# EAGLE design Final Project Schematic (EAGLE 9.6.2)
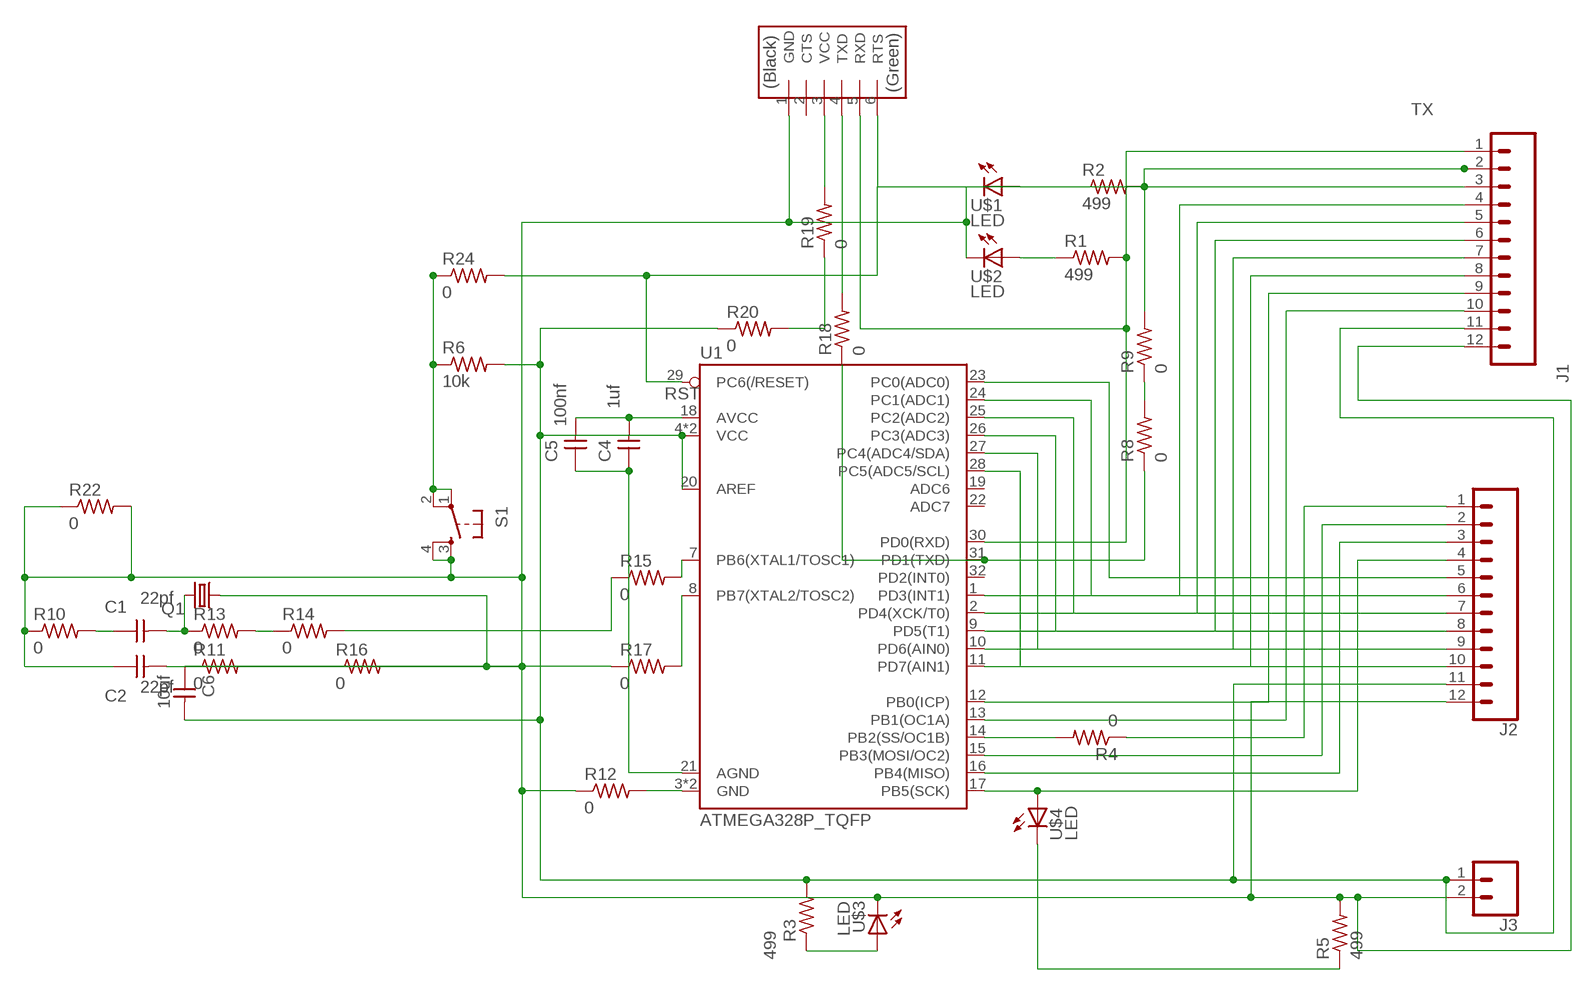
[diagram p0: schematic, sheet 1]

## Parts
C1  22pf  CAP_UNPOLARIZED  [C1206]
C2  22pf  CAP_UNPOLARIZED  [C1206]
C4  1uf  CAP_UNPOLARIZED  [C1206]
C5  100nf  CAP_UNPOLARIZED  [C1206]
C6  10uf  CAP_UNPOLARIZED  [C1206]
J1  CONN_12LONGPADS  [1X12_LONGPADS]
J2  CONN_12LONGPADS  [1X12_LONGPADS]
J3  CONN_02PTH3  [1X02_LONGPADS]
Q1  CRYSTALSM49  [SM49]
R1  499  R1206  [R1206]
R2  499  R1206  [R1206]
R3  499  R1206  [R1206]
R4  0  R1206FAB  [R1206FAB]
R5  499  R1206  [R1206]
R6  10k  R1206  [R1206]
R8  0  R1206FAB  [R1206FAB]
R9  0  R1206FAB  [R1206FAB]
R10  0  R1206FAB  [R1206FAB]
R11  0  R1206FAB  [R1206FAB]
R12  0  R1206FAB  [R1206FAB]
R13  0  R1206FAB  [R1206FAB]
R14  0  R1206FAB  [R1206FAB]
R15  0  R1206FAB  [R1206FAB]
R16  0  R1206FAB  [R1206FAB]
R17  0  R1206FAB  [R1206FAB]
R18  0  R1206FAB  [R1206FAB]
R19  0  R1206FAB  [R1206FAB]
R20  0  R1206FAB  [R1206FAB]
R22  0  R1206FAB  [R1206FAB]
R24  0  R1206FAB  [R1206FAB]
S1  SW_SWITCH_TACTILE_6MM6MM_SWITCH  [6MM_SWITCH]
U1  ATMEGA328P_TQFP  [TQFP32-08]
U$1  LED  [LED1206]
U$2  LED  [LED1206]
U$3  LED  [LED1206]
U$4  LED  [LED1206]
U$5  CONN_06_FTDI-SMD-HEADER  [1X06SMD]

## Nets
3: J1.4 U1.1(PD3(INT1))
4: J1.5 U1.2(PD4(XCK/T0))
5: J1.6 U1.9(PD5(T1))
6: J1.7 U1.10(PD6(AIN0))
7: J1.8 U1.11(PD7(AIN1))
8: J1.9 U1.12(PB0(ICP))
9: J1.10 U1.13(PB1(OC1A))
10: J2.1 R4.1
11: J2.2 U1.15(PB3(MOSI/OC2))
12: J2.3 U1.16(PB4(MISO))
13: J2.4 U1.17(PB5(SCK)) U$4.1(A)
A0: J2.5 U1.23(PC0(ADC0))
A1: J2.6 U1.24(PC1(ADC1))
A2: J2.7 U1.25(PC2(ADC2))
A3: J2.8 U1.26(PC3(ADC3))
A4: J2.9 U1.27(PC4(ADC4/SDA))
A5: J2.10 U1.28(PC5(ADC5/SCL))
GND [through pad 2]: C1.1 C2.1 C2.2 C4.1 C5.1 C6.1 J1.12 J2.12 J3.2 Q1.1 R5.2 R10.1 R10.2 R11.1 R12.1 R12.2 R22.1 R22.2 S1.3(S) S1.4(S1) U1.3(GND) U1.5(GND) U1.21(AGND) U$1.2(C) U$2.2(C) U$3.2(C) U$5.1(GND)
N$1: R4.2 U1.14(PB2(SS/OC1B))
N$2: R2.1 U$1.1(A)
N$18: R6.1 R24.1 S1.1(P) S1.2(P1)
N$25: R18.2 U$5.4(TXD)
N$26: R3.1 U$3.1(A)
N$27: C1.2 Q1.2 R13.1
N$28: R17.2 U1.8(PB7(XTAL2/TOSC2))
N$29: R5.1 U$4.2(C)
N$39: R15.2 U1.7(PB6(XTAL1/TOSC1))
N$40: R13.2 R14.1
N$41: R11.2 R16.1 R16.2 R17.1
N$42: R14.2 R15.1
RST [through pad 2]: J1.3 R24.2 U1.29(PC6(/RESET)) U$5.6(RTS)
RX: J1.1 R1.1 R1.2 U1.30(PD0(RXD)) U$2.1(A) U$5.5(RXD)
TX: J1.2 R2.2 R8.1 R8.2 R9.1 R9.2 R18.1 U1.31(PD1(TXD))
VCC [through pad 2]: C4.2 C5.2 C6.2 J1.11 J2.11 J3.1 R3.2 R6.2 R19.1 R19.2 R20.1 R20.2 U1.4(VCC) U1.6(VCC) U1.18(AVCC) U1.20(AREF) U$5.3(VCC)
Unconnected: U1.19(ADC6) U1.22(ADC7) U1.32(PD2(INT0)) U$5.2(CTS)

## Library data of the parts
C1 C2 C5 C6 = eagle_fab:CAP_UNPOLARIZED
C4 = eagle_fab:CAP_UNPOLARIZED; SPICEPREFIX: C
J1 J2 = SparkFun-Connectors:CONN_12: Multi connection point. Often used as Generic Header-pin footprint for 0.1 inch spaced/style header connections On any of the 0.1 inch spaced packages, you can populate with these: Break Away Headers - Straight (PRT-00116) Break Away Male Headers - Right Angle (PRT-00553) Female Headers (PRT-00115)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
J3 = SparkFun-Connectors:CONN_02: Multi connection point. Often used as Generic Header-pin footprint for 0.1 inch spaced/style header connections
Q1 = crystal:CRYSTAL: CRYSTAL; OC_FARNELL: unknown; OC_NEWARK: unknown
R1-R6 R8-R20 = eagle_fab:R: Resistor (US Symbol)
R22 R24 = fab_new:R: Resistor (US Symbol)
S1 = eagle_fab:SW_SWITCH_TACTILE_6MM: OMRON SWITCH
U1 = SparkFun-IC-Microcontroller:ATMEGA328P_TQFP: Popular 328P in QFP Storefront component: ATmega328 - TQFP (COM-13448) Datasheet SparkFun Products SparkFun RedBoard - Programmed with Arduino (DEV-12757) Arduino Pro Mini 328 - 5V/16MHz (DEV-11113) Arduino Pro Mini 328 - 3.3V/8MHz (DEV-11114) SparkFun OpenLog (DEV-13712) SparkFun MicroView - OLED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; PROD_ID: IC-09069
U$1-U$4 = eagle_fab:LED: LED
U$5 = eagle_fab:CONN_06_FTDI-SMD-HEADER

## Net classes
0 default: width 0.406 mm
1 ground: width 0.559 mm
2 vcc: width 0.559 mm
3 through pad: width 0.33 mm
4 bubble: width 0.229 mm
5 through pad 2: width 0.279 mm

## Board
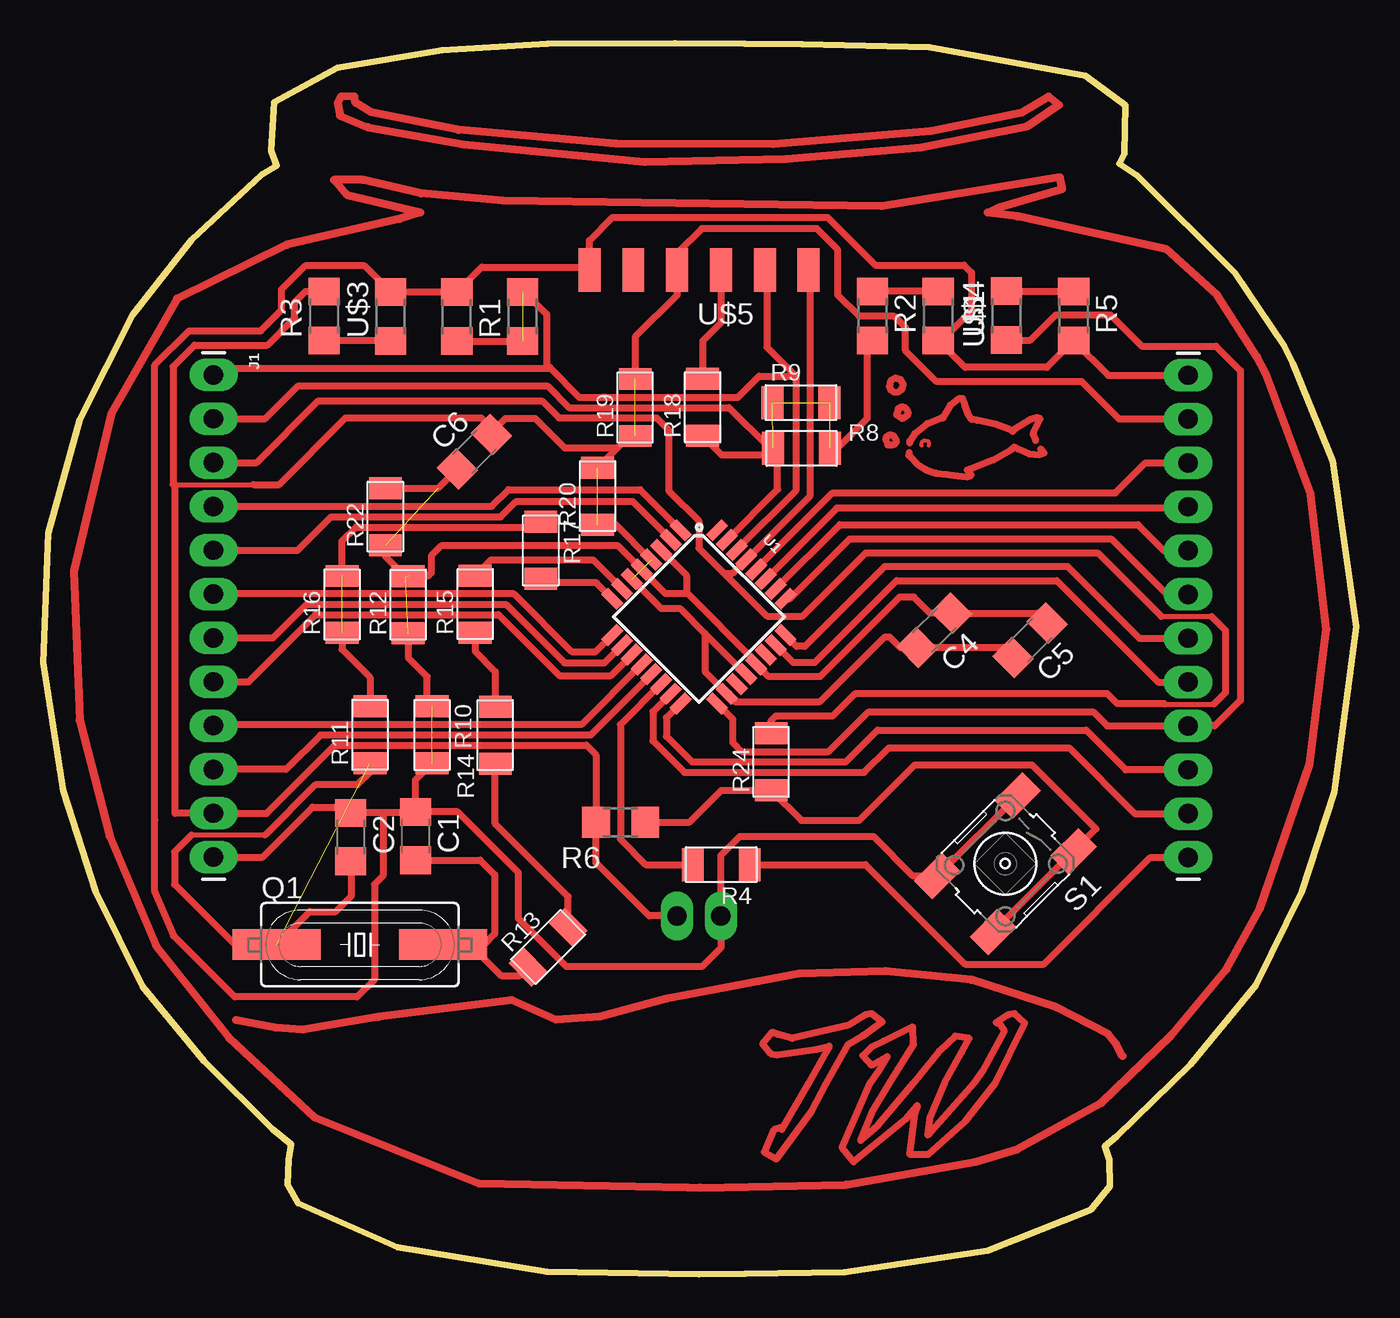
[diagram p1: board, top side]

Size 76.12 x 71.34 mm. Coordinates in mm from the lower left corner, seen from the top.
Outline: 40.67,71.3 36.62,71.34 29.24,71.32 23.12,70.94 17.08,69.91 13.39,67.93 13.22,65.12 13.55,64.24 12.66,63.71 8.62,59.94 5.19,55.61 2.12,49.51 0.29,42.93 0,35.44 1.15,28.03 3.04,22.18 5.77,16.68 9.33,12.35 13.31,8.41 14.38,7.53 14.24,6.64 14.16,5.19 14.77,4.13 20.53,1.58 29.21,0.16 38.03,0 40.67,0.04 46.44,0.14 54.74,1.38 60.74,3.76 61.83,5.1 61.8,6.64 61.55,7.42 62.22,8 66.51,12.14 70.29,16.74 72.96,22.17 74.84,27.93 76.12,37.52 74.75,47.11 72.44,52.79 71.92,53.84 69.07,58.03 63.42,63.66 62.38,64.35 62.68,64.93 62.73,67.74 60.4,69.45 51.37,71.1 43.99,71.27 40.67,71.3
Copper layers (1*16): Top 0.035mm / dielectric 1.5mm / Bottom 0.035mm
Design rules "OthermillDRC_30_deg_v2": minimum track width 6mil, minimum drill 0.8mm, track to track 6mil, track to pad 6mil, pad to pad 6mil, via to via 6mil, smd to smd 0mil, copper to edge 0mil, drill to drill 6mil, minimum pad ring 10mil, minimum via ring 10mil, stop-mask expansion 1mil, vias tented up to drill 30mil, thermal gap 6mil

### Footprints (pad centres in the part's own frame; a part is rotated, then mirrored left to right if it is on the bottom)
C1206 = smd 1.6 x 1.8: 1 -1.4,0; 2 1.4,0
1X12_LONGPADS = drill 1.118 pad 1.88 long: 1 0,0; 2 2.54,0; 3 5.08,0; 4 7.62,0; 5 10.16,0; 6 12.7,0; 7 15.24,0; 8 17.78,0; 9 20.32,0; 10 22.86,0; 11 25.4,0; 12 27.94,0
1X02_LONGPADS = drill 1.118 pad 1.88 long: 1 0,0; 2 2.54,0
SM49 = smd 5.08 x 1.778: 1 -4.826,0; 2 4.826,0
R1206 = smd 1.6 x 1.803: 1 -1.422,0; 2 1.422,0
R1206FAB = smd 1.27 x 1.905: 1 -1.651,0; 2 1.651,0
6MM_SWITCH = smd 2.286 x 1.524: 1 -3.302,2.286; 2 3.302,2.286; 3 -3.302,-2.286; 4 3.302,-2.286
TQFP32-08 = smd 1.27 x 0.559: 1 -4.293,2.8; 2 -4.293,2; 3 -4.293,1.2; 4 -4.293,0.4; 5 -4.293,-0.4; 6 -4.293,-1.2; 7 -4.293,-2; 8 -4.293,-2.8; 17 4.293,-2.8; 18 4.293,-2; 19 4.293,-1.2; 20 4.293,-0.4; 21 4.293,0.4; 22 4.293,1.2; 23 4.293,2; 24 4.293,2.8 | smd 0.559 x 1.27: 9 -2.8,-4.293; 10 -2,-4.293; 11 -1.2,-4.293; 12 -0.4,-4.293; 13 0.4,-4.293; 14 1.2,-4.293; 15 2,-4.293; 16 2.8,-4.293; 25 2.8,4.293; 26 2,4.293; 27 1.2,4.293; 28 0.4,4.293; 29 -0.4,4.293; 30 -1.2,4.293; 31 -2,4.293; 32 -2.8,4.293
LED1206 = smd 1.6 x 1.803: 1 -1.422,0; 2 1.422,0
1X06SMD = smd 2.54 x 1.27: 1 0,6.35; 2 0,3.81; 3 0,1.27; 4 0,-1.27; 5 0,-3.81; 6 0,-6.35

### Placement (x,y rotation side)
C1  21.58,25.4 270 top
C2  17.83,25.34 270 top
C4  51.67,37.32 225 top
C5  57.21,36.75 225 top
C6  25,47.67 45 top
J1  9.88,52.12 270 top
J2  66.37,24.16 90 top
J3  36.74,20.77 0 top
Q1  18.36,19.11 0 top
R1  27.79,55.51 90 top
R2  48.06,55.54 270 top
R3  16.28,55.54 90 top
R4  39.31,23.75 180 top
R5  59.73,55.53 270 top
R6  33.47,26.21 180 top
R8  43.96,47.86 0 top
R9  43.93,50.52 0 top
R10  22.54,31.26 270 top
R11  18.95,31.27 90 top
R12  21.16,38.81 90 top
R13  29.27,18.97 45 top
R14  26.21,31.25 90 top
R15  25.04,38.84 90 top
R16  17.32,38.82 90 top
R17  28.85,41.95 270 top
R18  38.22,50.24 90 top
R19  34.32,50.23 90 top
R20  32.14,45.09 90 top
R22  19.84,43.91 90 top
R24  42.2,29.7 90 top
S1  55.77,23.8 225 top
U1  38.01,38.1 315 top
U$1  51.88,55.54 270 top
U$2  23.98,55.5 90 top
U$3  20.14,55.51 90 top
U$4  55.83,55.56 90 top
U$5  38.02,58.2 90 top

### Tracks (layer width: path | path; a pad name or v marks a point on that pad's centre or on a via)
3
  Top 0.406: J1.4 26,44.5 26.97,45.47 34.6,45.47 U1.1
4
  Top 0.406: J1.5 14.75,41.96 16.69,43.9 26.53,43.9 27.42,44.79 34.17,44.79 36.39,42.57 U1.2
5
  Top 0.406: J1.6 27.29,39.43 30.64,36.08 32.03,36.08 U1.9
6
  Top 0.406: J1.7 13.33,36.88 15.28,38.83 26.83,38.83 30.22,35.44 32.54,35.44 33.56,36.46 U1.10
7
  Top 0.406: J1.8 11.91,34.34 15.79,38.23 26.39,38.23 29.92,34.7 32.91,34.7 U1.11
8
  Top 0.406: U1.12 31.21,31.86 9.94,31.86 J1.9
9
  Top 0.406: U1.13 31.73,31.26 16.07,31.26 14.08,29.26 J1.10
10
  Top 0.406: J2.1 66.34,24.16 64.19,24.16 58.01,17.98 53.43,17.98 47.67,23.75 R4.1
11
  Top 0.406: U1.15 35.35,32.61 35.35,30.91 37.17,29.08 47.59,29.08 49.01,30.5 59.47,30.5 63.27,26.7 J2.2
12
  Top 0.406: U1.16 36.13,32.26 36.13,31.18 37.61,29.69 46.52,29.69 48.36,31.54 60.45,31.54 62.75,29.24 J2.3
13
  Top 0.406: U$4.1 57.23,54.14 58.7,55.6 61.86,55.6 63.67,53.79 67.97,53.79 69.39,52.37 69.39,33.27 67.91,31.78 J2.4 61.68,31.78 60.86,32.6 47.84,32.6 45.53,30.29 40.49,30.29 39.96,30.82 39.96,32.19 U1.17 39.06,33.07
A0
  Top 0.406: U1.23 43.47,35.47 44.73,35.47 49.46,40.2 58.75,40.2 64.64,34.32 J2.5
A1
  Top 0.406: U1.24 43.68,36.39 44.15,36.39 48.79,41.02 59.38,41.02 63.54,36.86 J2.6
A2
  Top 0.406: U1.25 43.29,39.15 46.76,42.62 61.92,42.62 65.14,39.4 J2.7
A3
  Top 0.406: U1.26 46.18,43.44 63.46,43.44 64.96,41.94 J2.8
A4
  Top 0.406: U1.27 46,44.39 66.28,44.39 J2.9
A5
  Top 0.406: U1.28 45.75,45.28 62.15,45.28 63.89,47.02 J2.10
GND  (5 unrouted)
  Top 0.279: 12.87,25.45 8.6,25.45 | 17.85,23.91 C2.2
  Top 0.406: J2.12 61.74,52.1 R5.2 58.18,52.56 53.44,52.56 51.99,54.01 | 51.99,54.01 U$1.2 | 20.18,56.92 U$2.2 25.42,58.36 31.51,58.36 U$5.1 31.67,59.9 33.01,61.24 45.46,61.24 48.23,58.48 53.38,58.48 53.81,58.05 53.81,55.83 51.99,54.01 | U$3.2 19.57,56.92 19.49,56.84 | S1.3 S1.4 50.43,23.08 48.15,25.36 40.36,25.36 39.28,24.28 J3.2 39.28,18.92 38.19,17.83 30.34,17.83 27.55,20.62 27.55,23.28 24.03,26.8 C1.1 | J1.12 12.73,24.18 15.62,27.07 17.5,27.07 C2.1 | C1.1 21.58,28.65 R10.2 | C2.1 17.83,27.07 | C1.1 21.52,26.74 19.69,26.74 | 19.69,26.74 C2.1 | R12.1 21.16,35.74 22.26,34.64 22.26,33.19 R10.1 22.49,32.96 | U$3.2 18.63,58.44 15.19,58.44 13.81,57.06 13.81,55.87 12.61,54.68 8.45,54.68 6.48,52.7 6.48,26.34 | 21,40.43 19.84,41.6 R22.1 | R22.2 22.89,45.56 C6.1 | R12.2 22.3,40.46 22.49,40.65 22.49,41.63 23.07,42.21 33.33,42.21 U1.5 34.69,40.83 36.06,39.46 37.29,39.46 37.29,40.51 U1.3 | C2.2 17.16,23.94 | R11.1 18.95,29.1 18.21,28.36 15.78,28.36 12.87,25.45 | 6.48,26.34 6.46,26.36 | U$3.2 | U$3.2 20.18,56.92 | U$3.2 20.17,56.93 20.18,56.92 | 8.6,25.45 7.62,24.48 7.62,22.6 11.12,19.11 Q1.1 15.45,21.03 16.96,21.03 17.85,21.92 17.85,23.91 | 19.69,26.74 19.69,23.1 19.2,22.61 19.2,17.09 18.19,16.08 11.11,16.08 7.57,19.61 6.48,22.18 6.48,26.34 | C5.1 57.63,38.31 C4.1 51.41,38.31 50.48,39.24 50.48,39.25 49.63,39.25 45.03,34.64 42.05,34.64 41.35,35.35 U1.21 41.33,35.47 37.31,39.49
N$1
  Top 0.406: U1.14 33.46,31.85 33.46,25.22 34.92,23.75 R4.2
N$2
  Top 0.406: U$1.1 R2.1
N$18
  Top 0.406: S1.2 S1.1 61.02,25.82 57.32,29.53 50.53,29.53 47.31,26.31 43.94,26.31 R24.1 39.31,28.05 37.48,26.21 R6.1 34.93,26.25
N$25
  Top 0.406: 39.29,58.12 U$5.4 39.29,55.14 38.22,54.07 R18.2
N$26
  Top 0.406: R3.1 20.11,54.12 U$3.1
N$27
  Top 0.406: C1.2 25.34,24 26.18,23.16 26.18,19.74 25.55,19.11 Q1.2 24.76,19.11 26.55,17.32 27.62,17.32 R13.1
N$28
  Top 0.406: U1.8 32.09,40.06 32.09,40.07 29.08,40.07 R17.2
N$29
  Top 0.406: R5.1 55.86,56.95 U$4.2
N$34
  Top 0.457: 62.57,12.65 62.18,13.36 61.72,13.94 58.74,15.48 53.8,17.07 48.82,17.57 43.82,17.43 37.38,16.21 36.15,15.97 32.27,14.94 29.71,14.77 27.15,15.9 19.47,14.92 15.06,14.18 13.47,14.3 11.18,14.74
N$35
  Top 0.457: 17.29,68.26 17.08,67.9 17.2,67.14 18.82,66.48 24.36,65.48 34.86,64.47 43.07,64.64 50.9,65.3 57.04,66.54 58.88,67.76 58.29,68.24 56.73,67.32 51.44,66.25 42.33,65.5 33.19,65.51 24.08,66.31 19.01,67.35 18.12,67.88 18.03,68.24 17.29,68.26
N$36
  Top 0.457: 37.38,5.04 25.25,5.28 15.75,9.1 10.77,13.71 10.31,14.3 6.57,19.02 3.86,25.4 2.11,32.1 1.79,40.73 3.95,49.88 7.76,56.54 14.12,59.65 20.69,61.16 21.87,61.54 17.6,62.56 16.86,63.42 18.52,63.42 21.89,62.64 26.66,62.22 48.61,61.9 58.94,63.57 59.06,62.89 55.4,61.82 54.75,61.52 56.47,61.31 65.1,59.41 68.06,56.72 70.35,53.18 70.84,52.24 73.47,45.18 74.38,37.38 73.41,29.59 70.53,21.2 68.58,17.68 65.38,13.87 61.35,9.95 56.45,7.25 54.03,6.53 46.53,5.21 38.08,5.03 37.38,5.04 | 37.38,5.04
N$37
  Top 0.406: 49.06,48.65 48.87,48.53 48.82,48.36 48.96,48.06 49.29,48.08 49.4,48.16 49.45,48.34 49.3,48.57 49.06,48.65
N$38
  Top 0.406: 49.75,50.27 49.56,50.16 49.47,49.81 49.81,49.58 50.1,49.79 50.11,49.81 50.15,49.95 50,50.19 49.75,50.27
N$39
  Top 0.406: R15.2 25.95,41.4 31.88,41.4 U1.7
N$40
  Top 0.406: R13.2 30.43,21.89 26.21,26.12 R14.1
N$41  (1 unrouted)
  Top 0.406: R16.1 17.32,36.22 18.95,34.6 R11.2 | R16.2 17.32,42.5 18.13,43.3 28.55,43.3 R17.1
N$42
  Top 0.406: R15.1 25.04,36.1 26.21,34.93 R14.2
N$45
  Top 0.406: 48.01,15.11 47.66,15.05 46.68,14.45 43.41,13.68 42.56,13.91 42.24,14.02 41.7,13.37 42.16,12.8 42.53,12.73 44.83,13.05 45.57,13.22 45.41,12.92 44.51,11.33 44.37,11.07 42.8,8.39 42.73,8.51 42.37,8.38 41.81,7.09 42.49,6.68 44.52,9.42 45.39,11.07 46.68,13.34 47.51,13.84 48.62,14.63 48.01,15.11 | 48.01,15.11
N$49
  Top 0.406: 56.3,15.11 55.93,15.05 55.23,14.59 55.42,14.55 55.71,14.11 54.45,11.77 53.94,11.07 51.28,8.07 51.44,9.16 52.25,11.07 53.24,12.86 53.68,13.68 52.86,13.81 51.95,12.94 50.44,11.07 48.4,8.65 47.38,7.77 48.04,9.41 49.04,11.07 50.45,13.32 50.41,14.34 48.73,13.52 48,13.15 47.51,12.68 48.01,12.13 48.93,12.64 48.42,11.77 47.93,11.07 46.31,7.34 46.97,6.52 49.97,8.99 50.67,9.8 50.5,9.32 50.21,6.97 51.31,6.95 53.48,8.89 55.18,11.07 56.9,14.56 56.3,15.11
N$50
  Top 0.406: 50.19,47.62 50.18,47.46 50.69,46.92 51.18,46.63 51.75,46.43 52.37,46.36 53,46.27 53.55,46.21 53.79,46.31 53.68,46.49 53.57,46.61 53.71,46.66 55.08,47.2 56.14,47.82 56.29,47.95 56.48,47.83 57.15,47.55 57.77,47.5 58.01,47.61 57.83,47.83
N$51
  Top 0.229: 50.92,48.04 50.9,48.06 50.94,48.24 51.09,48.33 51.28,48.3 51.35,48.13 51.33,48.04
N$53
  Top 0.406: 49.4,51.94 49.12,51.78 49.04,51.46 49.14,51.25 49.31,51.13 49.57,51.14 49.78,51.29 49.83,51.46 49.86,51.58 49.7,51.84 49.4,51.94
N$54
  Top 0.406: 50.23,48.18 50.24,48.28 50.52,48.72 51.24,49.3 52.02,49.6 52.16,49.64 52.24,49.78 52.58,50.37 53.04,50.73 53.3,50.74 53.42,50.38 53.64,49.81 53.82,49.54 54.14,49.49 55.2,49.26 55.96,48.98 56.2,48.85 56.35,49 57.2,49.53 57.61,49.65 57.8,49.58 57.62,49.23 57.41,48.82 57.39,48.67 57.53,48.32
RST
  Top 0.279: 64.8,38.14 67.72,38.14 | 64.91,33.05 64.99,33.05 67.86,33.05
  Top 0.406: 44.24,58.2 U$5.6 44.45,58.12 44.45,45.1 U1.29 39.97,40.63 39.47,40.63 | J1.3 12.37,47.04 15.95,50.62 28.91,50.62 29.89,49.63 35.56,49.63 36.26,48.93 36.26,45.41 38.01,43.66 38.01,42.09 39.47,40.63 | 39.47,40.63 41.96,38.14 44.02,38.14 47.69,41.81 61.13,41.81 64.8,38.14 | 67.72,38.14 68.54,37.31 68.54,33.73 67.86,33.05 | 64.99,33.05 64.97,33.07 62.26,33.07 61.66,33.67 47.09,33.67 45.78,32.36 42.48,32.36 42.2,32.08 R24.2
RX  (1 unrouted)
  Top 0.406: 43.62,52.05 43.62,45.41 U1.30 | J1.1 10.26,52.5 29.4,52.5 | 43.62,52.05 41.49,52.05 40.27,50.82 31.07,50.82 29.4,52.5 | 29.4,52.5 29.19,52.71 29.19,55.64 27.9,56.93 R1.2 | U$2.1 27.78,54.08 R1.1 | U$5.5 41.95,58.08 41.95,53.73 43.62,52.05
TX  (3 unrouted)
  Top 0.406: U1.31 42.57,45.49 42.57,47.49 42.31,47.49 | 42.31,47.49 R8.1 42.12,47.86 39.75,50.23 30.48,50.23 29.23,51.48 14.78,51.48 12.88,49.58 J1.2 | R9.2 45.61,50.48 | R18.1 39.33,47.49 42.31,47.49 | R8.2 46.04,47.86 47.76,49.58 47.76,53.82 R2.2
VCC  (3 unrouted)
  Top 0.279: 7.65,45.77 12.19,45.77
  Top 0.356: 7.54,45.77 7.65,45.77
  Top 0.406: J2.11 62.37,49.56 60.2,51.73 51.78,51.73 49.98,53.53 49.98,54.87 49.35,55.51 47.31,55.51 46.07,56.75 46.07,59.37 44.84,60.59 38.18,60.59 36.75,59.16 U$5.3 36.75,56.75 34.32,54.32 R19.2 | J3.1 35.13,20.77 32.05,23.85 R6.2 32.05,30.11 31.49,30.66 16.9,30.66 12.96,26.72 J1.11 7.65,26.72 7.65,45.77 | R3.2 15.21,56.96 14.59,56.34 14.59,55.42 13.01,53.84 8.78,53.84 7.54,52.6 7.54,45.77 | C6.2 26.37,48.66 | 35.22,41.45 U1.4 | 32.57,43.01 R20.1 32.16,43.47 33.17,43.47 35.19,41.45 35.22,41.45 | 35.23,41.45 35.22,41.45 | 12.19,45.77 13.67,45.77 17.53,49.63 25.4,49.63 26.12,48.91 | 26.12,48.91 26.37,48.66 | 26.37,48.66 26.59,48.44 | U1.6 35.82,38.59 36.91,38.59 38.37,37.13 | 39.76,33.65 U1.18 | 55.89,35.73 56.2,35.73 C5.2 55.65,36.33 C4.2 49.67,36.33 49.06,36.94 48.79,36.94 45.04,33.19 40.09,33.19 U1.18 | U1.18 38.37,34.91 38.37,37.13 | R20.2 33.26,47.87 | 33.26,47.87 33.97,48.58 R19.1 | 33.26,47.87 30.25,47.87 28.54,49.58 26.79,49.58 26.12,48.91 | U1.20 40.72,34.78 38.37,37.13

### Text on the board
bottom_silk: FishBowl V2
